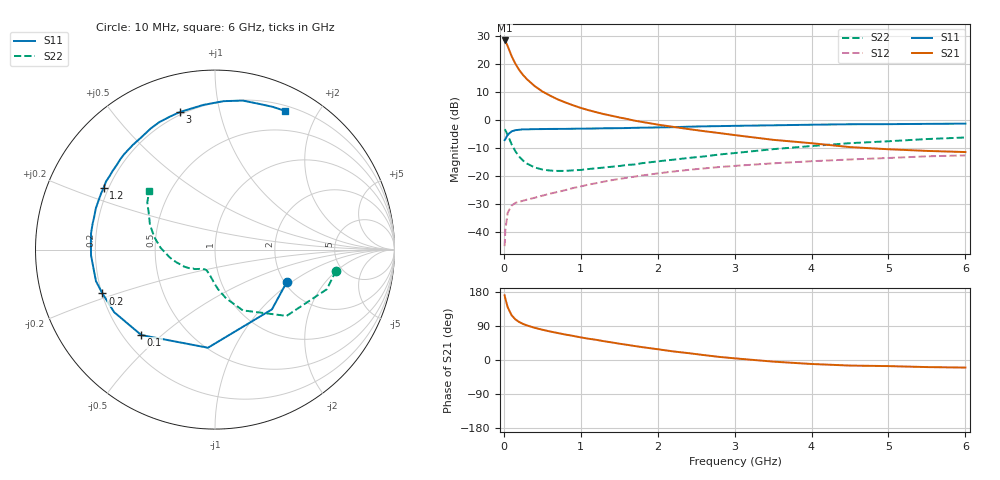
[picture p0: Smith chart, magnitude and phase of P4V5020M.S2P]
! SIEMENS Small Signal Semiconductors
! BFP182
! Si NPN RF Bipolar Junction Transistor in SOT143
! VCE = 0.5 V  IC = 20 mA
! Common Emitter S-Parameters:  March  1996
# GHz  S  MA  R  50
!  f  S11  S21  S12  S22
! GHz  MAG  ANG  MAG  ANG  MAG  ANG  MAG  ANG
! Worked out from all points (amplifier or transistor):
!   36 points, 10 MHz to 6 GHz, reference 50 ohm
!   highest |S21| = 28.5 dB at 10 MHz (marker M1)
!   |S21| within 3 dB of that: start of sweep to 63.88 MHz
!   unconditionally stable (mu >= 1): start of sweep to 15.49 MHz; 218.6 MHz to end of sweep
!   at 250 MHz: K = 1.10, MAG = 20.6 dB, |S12| = -28.8 dB
!   at 1.4 GHz: K = 2.39, MAG = 4.9 dB, |S12| = -21.5 dB
!   at 6 GHz: K = 1.86, MAG = -4.8 dB, |S12| = -12.6 dB
!   S11 on the Smith chart (normalised r, x): 10 MHz: 2.06, -0.92; 100 MHz: 0.27, -0.43; 200 MHz: 0.20, -0.18; 1.2 GHz: 0.18, +0.25; 3 GHz: 0.19, +0.76; 6 GHz: 0.26, +1.60
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0.01  0.4391 -24.1  26.53 170.6  0.0056 75.5  0.685 -9.8
0.02  0.4599 -46.4  25.78 161.8  0.011 71.9  0.6612 -19.5
0.05  0.5482 -94.1  21.01 139.3  0.0221 54.8  0.5437 -42.8
0.1  0.6288 -130.8  14.04 118.3  0.0297 38.1  0.3725 -65.4
0.15  0.6613 -148.2  10.18 107.2  0.0333 33.5  0.2783 -77.2
0.2  0.6732 -158.7  7.858 100.1  0.0348 31.8  0.2228 -85.3
0.25  0.6859 -165.1  6.406 95.2  0.0363 32.1  0.189 -91.1
0.3  0.6847 -170.2  5.385 91.3  0.038 33.3  0.1681 -95.0
0.4  0.6914 -177.4  4.066 85.0  0.041 35.8  0.1428 -102.2
0.5  0.6924 177.1  3.257 79.9  0.0447 38.4  0.1312 -107.7
0.6  0.6965 172.4  2.748 75.3  0.0485 40.5  0.1257 -111.4
0.7  0.697 168.1  2.349 71.2  0.0522 42.5  0.1238 -114.4
0.9  0.7025 161.0  1.841 63.6  0.0613 44.8  0.1267 -120.6
1.1  0.7073 153.9  1.508 56.2  0.0706 45.9  0.1338 -126.1
1.2  0.7097 151.0  1.388 53.3  0.0747 46.0  0.138 -128.9
1.7  0.7294 136.2  0.979 36.9  0.0979 44.7  0.1616 -139.4
2.2  0.7482 123.3  0.759 22.7  0.1206 40.9  0.1963 -151.2
3  0.791 104.3  0.541 4.4  0.1523 32.7  0.2581 -170.9
3.5  0.8086 94.7  0.445 -4.3  0.1692 27.4  0.303 178.2
4.5  0.8447 79.4  0.33 -14.7  0.1982 16.9  0.3879 159.1
5.5  0.8576 68.1  0.282 -18.7  0.2255 7.2  0.4594 145.2
6  0.8661 63.1  0.269 -20.0  0.2345 1.8  0.49 138.5
